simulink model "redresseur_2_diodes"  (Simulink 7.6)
settings: Solver=ode23tb  StartTime=0.0  StopTime=0.2  RelTol=1e-3
InitFcn:
  | clear all
  | close all
  | clc
  | delete *.mat
StopFcn:
  | close all
  | load v1_v2.mat
  | plot(x(1,:),x(2,:),x(1,:),x(3,:))
  | grid
  | title('Tension du primaire et de sortie')
  | xlabel('temps')
  | axis([0 0.05 -250 250])
  | 
  | figure
  | 
  | load i1_i2.mat
  | plot(y(1,:),y(2,:),y(1,:),y(3,:))
  | grid
  | title('Courant du primaire et de sortie')
  | xlabel('temps')
  | axis([0 0.05 -2 3.5])
libraries: powerlib x15

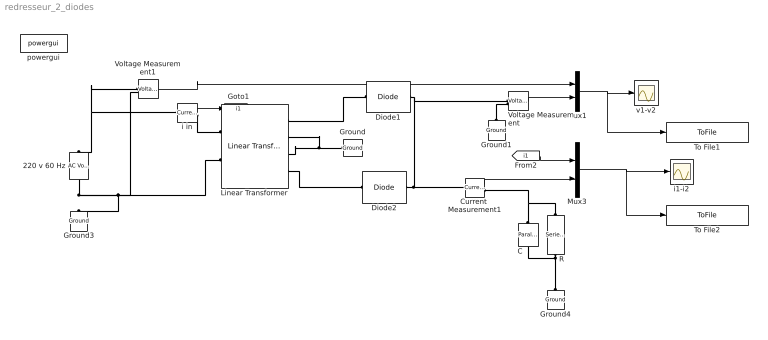
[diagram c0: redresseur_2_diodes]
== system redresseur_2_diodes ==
  220 v 60 Hz : powerlib/Electrical Sources/AC Voltage Source  Description=source block  DialogController=POWERSYS.PowerSysDialog  SystemSampleTime=-1  Amplitude=220  Phase=0  Frequency=60  SampleTime=0  Measurements=None
  C : powerlib/Elements/Parallel RLC Branch  DialogController=POWERSYS.PowerSysDialog  PhysicalDomain=powersysdomain  SubClassName=unknown  LeftPortType=p1  RightPortType=p1  LConnTagsString=a  RConnTagsString=__new0  BranchType=C  Resistance=1  Inductance=1e-3  SetiL0=off  InitialCurrent=0  Capacitance=250e-6  Setx0=off  InitialVoltage=0  Measurements=None
  Current  Measurement1 : powerlib/Measurements/Current Measurement  DialogController=POWERSYS.PowerSysDialog  SystemSampleTime=-1  PhasorSimulation=off  OutputType=Complex  PSBequivalent=0
  Diode1 : powerlib/Power Electronics/Diode  DialogController=POWERSYS.PowerSysDialog  SystemSampleTime=-1  Ron=0.001  Lon=0  Vf=0.8  IC=0  UseSnubber=off  Rs=500  Cs=250e-9  Measurements=off
  Diode2 : powerlib/Power Electronics/Diode  DialogController=POWERSYS.PowerSysDialog  SystemSampleTime=-1  Ron=0.001  Lon=0  Vf=0.8  IC=0  UseSnubber=off  Rs=500  Cs=250e-9  Measurements=off
  Ground{,1,3..4} (4 alike) : powerlib/Elements/Ground  DialogController=POWERSYS.PowerSysDialog  PhysicalDomain=powersysdomain  SubClassName=unknown  LeftPortType=p1  RightPortType=p1  LConnTagsString=a
  Linear Transformer : powerlib/Elements/Linear Transformer  DialogController=POWERSYS.PowerSysDialog  PhysicalDomain=powersysdomain  SubClassName=unknown  LeftPortType=p1  RightPortType=p1  LConnTagsString=a|b  RConnTagsString=A|B|C|D  UNITS=SI  NominalPower=[75e3,60]  winding1=[120 27.648 0.22002]  winding2=[120 0.00384 0]  ThreeWindings=on  winding3=[120 0.00384 0]  RmLm=[1.3824e+005 366.69]  Measurements=None  DataType=on
  Mux1 : Mux  Inputs=2
  Mux3 : Mux  Inputs=2
  R : powerlib/Elements/Series RLC Branch  DialogController=POWERSYS.PowerSysDialog  PhysicalDomain=powersysdomain  SubClassName=unknown  LeftPortType=p1  RightPortType=p1  LConnTagsString=__new0  RConnTagsString=__new0  BranchType=R  Resistance=1e3  Inductance=1e-3  SetiL0=off  InitialCurrent=0  Capacitance=1e-6  Setx0=off  InitialVoltage=0  Measurements=None
  To File1 : ToFile  Filename=v1_v2  MatrixName=x
  To File2 : ToFile  Filename=i1_i2  MatrixName=y
  Voltage Measurement : powerlib/Measurements/Voltage Measurement  DialogController=POWERSYS.PowerSysDialog  SystemSampleTime=-1  PhasorSimulation=off  OutputType=Complex  PSBequivalent=0
  Voltage Measurement1 : powerlib/Measurements/Voltage Measurement  DialogController=POWERSYS.PowerSysDialog  SystemSampleTime=-1  PhasorSimulation=off  OutputType=Complex  PSBequivalent=0
  i in : powerlib/Measurements/Current Measurement  Tag=PoWeRsYsTeMmEaSuReMeNt  DialogController=POWERSYS.PowerSysDialog  SystemSampleTime=-1  PhasorSimulation=off  OutputType=Magnitude  PSBequivalent=0
  i1-i2 : Scope
  powergui : powerlib/powergui  SystemSampleTime=-1  SimulationMode=Continuous  SampleTime=0  frequency=60  SPID=off  DisableSnubberDevices=off  DisableRonSwitches=off  DisableVfSwitches=off  SwTol=0  Interpol=off  frequencyindice=60  echomessages=off  HookPort=off  DisplayEquations=off  FunctionMessages=off  EnableUseOfTLC=off  x0status=blocks  RestoreLinks=warning  ResistiveCurrentMeasurement=off  Frange=[0:2:500]  Ylog=off  Xlog=on  ShowGrid=off  save=off  variable=ZData  ZoomFFT=on  StartTime=0.0  cycles=1  DisplayStyle=1  fundamental=60  FreqAxis=off  MaxFrequency=1000  frequencyindicesteady=1  RmsSteady=1  display=off  Ts=0  methode=off
  v1-v2 : Scope
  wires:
  i in/1 -> [i1]
  Voltage Measurement/1 -> Mux1/2
  Voltage Measurement1/1 -> Mux1/1
  Mux1/1 -> v1-v2/1, To File1/1
  Current  Measurement1/1 -> Mux3/2
  [i1] -> Mux3/1
  Mux3/1 -> i1-i2/1, To File2/1
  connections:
  Ground/LConn1 -- Linear Transformer/RConn2 -- Linear Transformer/RConn3
  i in/RConn1 -- Linear Transformer/LConn1
  220 v 60 Hz/LConn1 -- Ground3/LConn1 -- Linear Transformer/LConn2 -- Voltage Measurement1/LConn2
  Diode1/RConn1 -- Current  Measurement1/LConn1 -- Diode2/RConn1 -- Voltage Measurement/LConn1
  Linear Transformer/RConn1 -- Diode1/LConn1
  Ground1/LConn1 -- Voltage Measurement/LConn2
  Linear Transformer/RConn4 -- Diode2/LConn1
  i in/LConn1 -- 220 v 60 Hz/RConn1 -- Voltage Measurement1/LConn1
  R/LConn1 -- Current  Measurement1/RConn1 -- C/LConn1
  R/RConn1 -- Ground4/LConn1 -- C/RConn1
